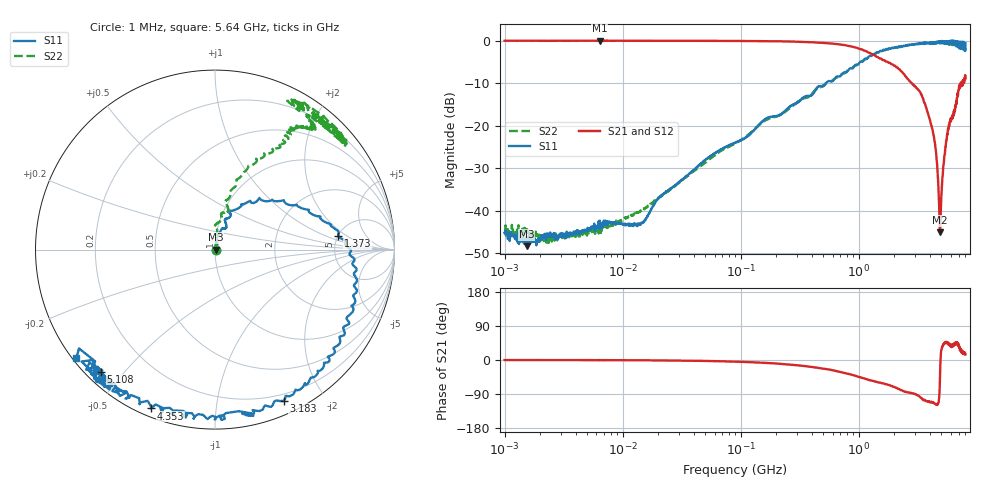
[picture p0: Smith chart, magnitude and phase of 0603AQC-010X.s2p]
!s-Parameter Generated by FASTRON Sdn. Bhd.
!FASTRON P/N : 0603AQC-010X
!Keysight Technologies: E5071C_MY46733604_B.14.02
!Date: Thu Jun 25 13:51:24 2026
!Version  :Rev00  Thu Jun 25 13:51:24 2026
!Data & Calibration Information:
!Freq  S11:SOLT2(ON)  S21:SOLT2(ON)  S12:SOLT2(ON)  S22:SOLT2(ON)
!PortZ  Port1:50+j0  Port2:50+j0
!When reading reference impedance value at option line is always used.
! Remarks : This data is being provided solely for informational purposes.
# Hz S dB R 50
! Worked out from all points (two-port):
!   1601 points, 1 MHz to 8 GHz, reference 50 ohm
!   highest |S21| = -0.01 dB at 6.4 MHz (marker M1); lowest = -45.0 dB at 4.884 GHz (marker M2)
!   |S21| within 3 dB of the highest: start of sweep to 1.26 GHz
!   lowest |S11| = -48.3 dB at 1.541 MHz (marker M3), VSWR 1.01, Z = 50.4 + j0.0233 ohm
!   |S11| at or under -10 dB: start of sweep to 528.5 MHz
!   |S22| runs from -47.6 to -0.3 dB; largest |S21 - S12| = 0.013
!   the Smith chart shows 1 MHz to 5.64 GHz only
!   S11 on the Smith chart (normalised r, x): 1 MHz: 1.01, +0.00; 1.373 GHz: 5.04, +1.45; 3.183 GHz: 0.13, -1.54; 4.353 GHz: 0.03, -0.67; 5.108 GHz: 0.04, -0.43; 5.64 GHz: 0.01, -0.34
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1000000  -45.20 0.4  -0.05 -0.1  -0.05 -0.1  -44.60 1.7
1541011  -48.30 3.5  -0.05 -0.2  -0.04 -0.1  -45.20 -6.7
2273910  -45.90 19.3  -0.04 -0.2  -0.05 -0.1  -46.60 25.5
4479405  -45.20 29.0  -0.05 -0.3  -0.05 -0.3  -45.10 34.5
6400096  -42.30 39.3  -0.01 -0.2  -0.01 -0.1  -42.80 32.6
1.449233e7  -42.80 52.0  -0.05 -0.8  -0.06 -0.8  -39.90 56.1
2.00676e7  -37.10 54.8  -0.06 -1.1  -0.06 -1.0  -37.00 72.4
8.994653e7  -24.00 81.1  -0.09 -4.4  -0.10 -4.3  -24.10 76.6
4.006501e8  -12.80 69.0  -0.38 -18.4  -0.38 -18.4  -12.60 71.7
8.377436e8  -6.57 35.9  -1.32 -37.4  -1.32 -37.5  -6.75 69.6
1.372751e9  -3.21 6.3  -3.54 -57.2  -3.56 -57.3  -3.10 57.4
1.7949e9  -1.93 -11.2  -5.23 -65.8  -5.25 -66.0  -1.90 57.0
2.398863e9  -1.21 -36.9  -7.80 -81.8  -7.83 -81.9  -1.27 51.8
3.183204e9  -0.67 -65.6  -11.50 -93.5  -11.50 -93.5  -0.80 55.1
3.771001e9  -0.47 -90.1  -16.30 -109.0  -16.30 -109.0  -0.59 47.3
4.352635e9  -0.41 -112.0  -23.10 -114.0  -23.10 -115.0  -0.64 50.1
4.88448e9  -0.43 -127.0  -45.00 -31.2  -45.20 -30.5  -0.44 44.0
5.108415e9  -0.63 -133.0  -32.20 35.4  -32.20 35.0  -0.55 46.7
5.64026e9  -0.18 -142.0  -22.10 44.8  -22.10 44.6  -0.62 59.6
6.110812e9  -0.36 -159.0  -18.30 33.9  -18.30 33.6  -0.86 48.9
6.72769e9  -0.13 -158.0  -14.90 44.4  -14.80 43.9  -0.66 75.0
8e9  -0.63 155.0  -8.87 14.6  -8.89 13.9  -1.67 68.9
